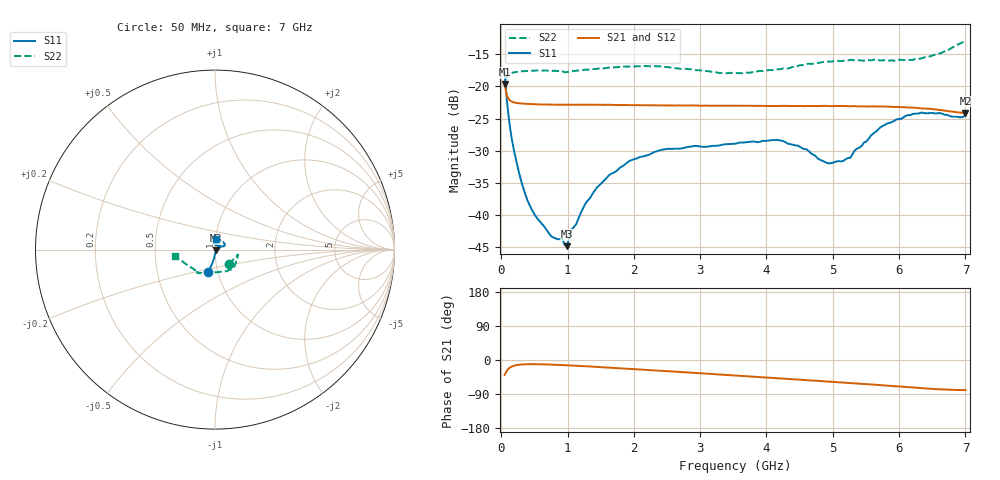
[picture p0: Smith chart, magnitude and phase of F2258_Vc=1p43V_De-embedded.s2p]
! Integrated Device Technology
! Corporate Headquarters
! 6024 Silver Creek Valley Road
! San Jose, CA 95138  USA
! Phone:  1-408-284-8200
! Toll Free:  1-800-223-1366
! Webpage:  http://www.idt.com/
! Timing and RF Division
! 515 Groton Road, Suite 102
! Westford, MA 01886-6024
! Device:  F2258
! Description: Voltage Variable RF Attenuator
! Frequency:  50.0 -  6000.00 MHz
! Package:  3x3 mm Thin QFN Plastic Package: 16 pin
! Ports:  2 RF, 2 DC
!  Pin  1  = NC
!  Pin  2  = NC
!  Pin  3  = RF2  = Port 2
!  Pin  4  = GND
!  Pin  5  = Vdd
!  Pin  6  = NC
!  Pin  7  = VCTRL
!  Pin  8  = NC
!  Pin  9  = GND
!  Pin 10  = RF1  = Port 1
!  Pin 11  = NC
!  Pin 12  = NC
!  Pin 13  = NC
!  Pin 14  = NC
!  Pin 15  = NC
!  Pin 16  = NC
! Vcntrl:  1.430 Volts
! Vdd:  +3.300 Volts
! Current:  1.161 mA
! Data:  The device was measured on a the F2258 evaluation board which has
!  individual transmission lines to the RF pins.  Data was collected
!  using a calibrated network analyzer.  The evaluation board was
!  de-embedded using a TRL calibration technique.
!  The reference plane is the edge of the package pin.
! Misc:  SN 10
!  Action Tracker AT0285
! Date Measured:  2014-12-10
! Date:  2016-01-13  MJV
! Note:
!  Integrated Device Technology supplies this data as a sample of measured
!  data at the package pin for this product.  Your particular data for this
!  product may vary.
!  Data was taken at 25 degrees C.
!  Integrated Device Technology reserves the right to change this data at anytime.
!Freq_(GHz)  S11M_(dB)  S11P_(deg)  S21M_(dB)  S21P_(deg)  S12M_(dB)  S12P_(deg)  S22M_(dB)  S22P_(deg)
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# GHz S dB R 50
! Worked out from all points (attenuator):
!   201 points, 50 MHz to 7 GHz, reference 50 ohm
!   highest |S21| = -19.69 dB at 50 MHz (marker M1); lowest = -24.1 dB at 7 GHz (marker M2)
!   lowest |S11| = -44.8 dB at 988.2 MHz (marker M3), VSWR 1.01, Z = 50.5 - j0.292 ohm
!   |S11| at or under -10 dB: start of sweep to end of sweep
!   |S22| runs from -19.2 to -12.8 dB; largest |S21 - S12| = 0.0005
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0.05  -17.78 -106.7  -19.69 -39.4  -19.69 -39.4  -19.16 -46.3
0.08475  -22.26 -100.7  -21.46 -27.5  -21.46 -27.5  -18.44 -23.9
0.15425  -27.94 -95.4  -22.33 -17.5  -22.34 -17.5  -17.90 -14.6
0.2585  -33.06 -89.0  -22.60 -12.7  -22.60 -12.7  -17.71 -12.0
0.36275  -36.80 -82.0  -22.70 -11.3  -22.71 -11.3  -17.60 -12.5
0.50175  -39.91 -66.8  -22.76 -11.0  -22.77 -11.0  -17.54 -14.2
0.745  -43.23 -41.0  -22.82 -12.1  -22.82 -12.1  -17.56 -18.8
0.91875  -43.61 -9.3  -22.84 -13.4  -22.83 -13.4  -17.60 -23.0
0.98825  -44.85 -30.4  -22.85 -13.9  -22.84 -13.9  -17.77 -24.2
1.05775  -42.32 -16.0  -22.84 -14.5  -22.84 -14.5  -17.65 -25.5
1.2315  -38.96 -0.3  -22.83 -16.1  -22.84 -16.1  -17.44 -28.9
1.6485  -33.62 11.3  -22.86 -20.5  -22.88 -20.5  -17.07 -36.8
1.9265  -31.63 20.5  -22.91 -23.4  -22.91 -23.4  -16.90 -41.8
2.37825  -29.97 32.4  -22.95 -28.1  -22.95 -28.2  -16.87 -50.5
3.525  -28.90 83.6  -22.99 -40.9  -22.97 -40.9  -17.95 -86.0
4.22  -28.42 102.7  -23.04 -48.8  -23.04 -48.8  -17.28 -110.7
4.7065  -30.61 91.8  -23.04 -54.3  -23.03 -54.3  -16.46 -120.2
4.94975  -31.98 72.4  -23.06 -57.1  -23.10 -57.0  -16.14 -122.4
5.15825  -31.58 51.7  -23.06 -59.7  -23.11 -59.6  -16.02 -124.2
5.85325  -25.68 22.0  -23.16 -68.1  -23.21 -67.9  -15.98 -131.0
6.33975  -24.05 29.4  -23.41 -74.3  -23.45 -74.2  -15.63 -143.4
7  -24.47 83.7  -24.14 -79.3  -24.16 -79.2  -12.84 -170.3
